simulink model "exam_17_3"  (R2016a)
settings: Solver=VariableStepAuto  StartTime=0.0  StopTime=10.0  RelTol=1e-3
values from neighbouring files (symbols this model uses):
  A = [1 2;3 4]    [exam_1_2.m]    (also in exam_1_7.m = 1.6; exam_10_12.m = 5; exam_10_20.m = [-0.5572,-0.7814;0.7814,0]; exam_11_10.m = [ones(1,30),zeros(1,N-29)])
  N = 21    [exam_10_11.m]    (also in exam_11_10.m = 60; exam_11_2.m = 0:15; exam_11_3_1.m = input('ÐòÁÐf1µÄ³¤¶ÈN='); exam_12_8.m = ceil(nn_1))
undefined symbols (not defined in the file or in its folder): constant, Torque
libraries: powerlib x11, powerlib_meascontrol x1, simulink x1

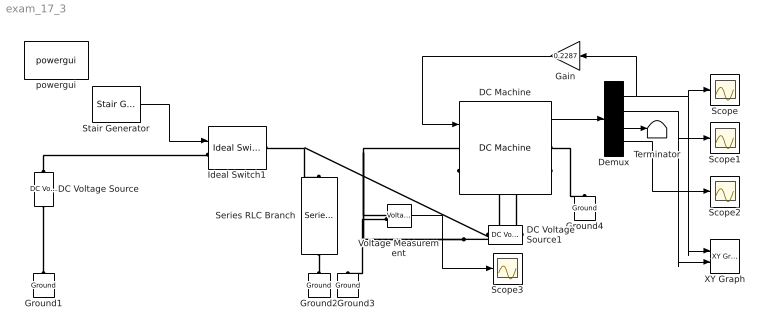
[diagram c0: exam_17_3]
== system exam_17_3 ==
  DC Machine : powerlib/Machines/DC Machine  PresetModel=No  MechanicalLoad=Torque TL  FieldType=Wound  ShowDetailedParameters=on  MeasurementBus=off  RLa="[ 0.6  0.012]"  RLf="[ 240  120]"  Laf=1.8  MachineConstant=Torque constant (N.m/A)  Ke=1.8  Kt=1.8  J=1  Bm=0  Tf=0  w0=1  Ifinit=1  TsPowergui=0  TsBlock=-1
  DC Voltage Source : powerlib/Electrical Sources/DC Voltage Source  Amplitude=240  Measurements=None
  DC Voltage Source1 : powerlib/Electrical Sources/DC Voltage Source  Amplitude=240  Measurements=None
  Demux : Demux
  Gain : Gain  Gain=0.2287
  Ground{1..4} (4 alike) : powerlib/Elements/Ground  LConnTagsString=a
  Ideal Switch1 : powerlib/Power Electronics/Ideal Switch  Ron=0  Lon=0  IC=0  Rs=inf  Cs=inf  Measurements=off
  Scope{,1..3} (4 alike) : Scope
  Series RLC Branch : powerlib/Elements/Series RLC Branch  LConnTagsString=__new0  RConnTagsString=__new0  BranchType=R  Resistance=10000  Inductance=0  SetiL0=off  InitialCurrent=0  Capacitance=inf  Setx0=off  InitialVoltage=0  Measurements=None
  Stair Generator : powerlib_meascontrol/Pulse & Signal Generators/Stair Generator  t=[0, 0.5]  e=[1, 1]  Ts=0
  Terminator : Terminator
  Voltage Measurement : powerlib/Measurements/Voltage Measurement  PhasorSimulation=off  OutputType=Complex  PSBequivalent=0
  XY Graph : simulink/Sinks/XY Graph  xmin=-1  xmax=1  ymin=-1  ymax=1  st=-1
  powergui : powerlib/powergui  Priority=1  SimulationMode=Continuous  SolverType=Tustin/Backward Euler (TBE)  SampleTime=50e-6  frequency=60  SPID=on  DisableSnubberDevices=off  DisableRonSwitches=off  DisableVfSwitches=off  SwTol=0  DisplayEquations=off  Interpol=off  ExternalGateDelay=off  methode=off  Ts=10  FunctionMessages=off  echomessages=off  HookPort=off  EnableUseOfTLC=off  x0status=blocks  frequencyindice=0  Pbase=100e6  ErrMax=1e-4  Iterations=50  UnitsV=kV  UnitsW=MW  buscounter=0  RestoreLinks=warning  ResistiveCurrentMeasurement=off  Frange=[0:2:500]  Ylog=off  Xlog=on  ShowGrid=off  save=off  variable=ZData  structure=0  ZoomFFT=off  StartTime=0.0  cycles=1  DisplayStyle=1  fundamental=60  FreqAxis=off  MaxFrequency=1000  frequencyindicesteady=1  RmsSteady=1  display=off
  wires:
  Demux/4 -> Scope2/1
  Stair Generator/1 -> Ideal Switch1/1
  DC Machine/1 -> Demux/1
  Demux/1 -> Gain/1, XY Graph/1, Scope/1
  Demux/2 -> XY Graph/2, Scope1/1
  Gain/1 -> DC Machine/1
  Voltage Measurement/1 -> Scope3/1
  Demux/3 -> Terminator/1
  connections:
  DC Voltage Source/RConn1 -- Ideal Switch1/LConn1
  Ideal Switch1/RConn1 -- DC Machine/LConn1 -- Voltage Measurement/LConn1 -- Series RLC Branch/LConn1
  Ground2/LConn1 -- Series RLC Branch/RConn1
  DC Voltage Source/LConn1 -- Ground1/LConn1
  Voltage Measurement/LConn2 -- Ground3/LConn1
  DC Voltage Source1/LConn1 -- DC Machine/RConn2
  DC Voltage Source1/RConn1 -- DC Machine/LConn2
  DC Machine/RConn1 -- Ground4/LConn1
